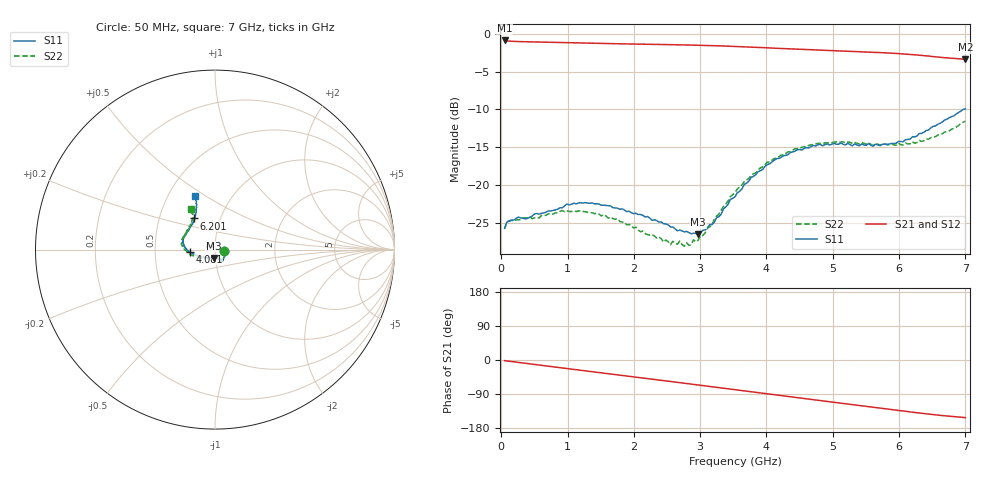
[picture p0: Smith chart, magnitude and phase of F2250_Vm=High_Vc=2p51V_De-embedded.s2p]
! Integrated Device Technology
! Corporate Headquarters
! 6024 Silver Creek Valley Road
! San Jose, CA 95138  USA
! Phone:  1-408-284-8200
! Toll Free:  1-800-223-1366
! Webpage:  http://www.idt.com/
! Timing and RF Division
! 515 Groton Road, Suite 102
! Westford, MA 01886-6024
! Device:  F2250
! Description: Voltage Variable RF Attenuator
! Frequency:  50.0 -  6000.00 MHz
! Package:  3x3 mm Thin QFN Plastic Package: 16 pin
! Ports:  2 RF, 3 DC
!  Pin  1  = GND
!  Pin  2  = NC
!  Pin  3  = RF1  = Port 1
!  Pin  4  = NC
!  Pin  5  = GND
!  Pin  6  = GND
!  Pin  7  = GND
!  Pin  8  = GND
!  Pin  9  = NC
!  Pin 10  = RF2  = Port 2
!  Pin 11  = NC
!  Pin 12  = GND
!  Pin 13  = GND
!  Pin 14  = VCNTRL
!  Pin 15  = VDD
!  Pin 16  = VMODE
! Vcntrl:  2.510 Volts
! Vmode:  +3.300 Volts
! Vdd:  +3.30  Volts
! Current:  1.314 mA
! Data:  The device was measured on a the F2250 evaluation board which has
!  individual transmission lines to the RF pins.  Data was collected
!  using a calibrated network analyzer.  The evaluation board was
!  de-embedded using a TRL calibration technique.
!  The reference plane is the edge of the package pin.
! Misc:  SN 10
!  Action Tracker AT0258
! Date Measured:  2014-11-26
! Date:  2015-10-15  MJV
! Note:
!  Integrated Device Technology supplies this data as a sample of measured
!  data at the package pin for this product.  Your particular data for this
!  product may vary.
!  Data was taken at 25 degrees C.
!  Integrated Device Technology reserves the right to change this data at anytime.
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# GHz S dB R 50
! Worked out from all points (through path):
!   201 points, 50 MHz to 7 GHz, reference 50 ohm
!   highest |S21| = -0.89 dB at 50 MHz (marker M1); lowest = -3.4 dB at 7 GHz (marker M2)
!   group delay of S21, straight-line fit = 61.2 ps
!   lowest |S11| = -26.5 dB at 2.969 GHz (marker M3), VSWR 1.10, Z = 49.1 - j4.62 ohm
!   |S11| at or under -10 dB: start of sweep to 6.967 GHz
!   |S22| runs from -28.1 to -11.6 dB; largest |S21 - S12| = 0.002
!   S11 on the Smith chart (normalised r, x): 50 MHz: 1.11, -0.02; 4.081 GHz: 0.75, -0.02; 6.201 GHz: 0.75, +0.27; 7 GHz: 0.68, +0.45
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0.05  -25.65 -10.7  -0.89 -1.8  -0.89 -1.8  -25.82 -10.9
0.1195  -24.75 -10.3  -0.98 -3.2  -0.98 -3.2  -24.68 -8.9
0.57125  -23.83 -31.3  -1.10 -13.3  -1.10 -13.3  -24.33 -31.4
0.91875  -23.00 -50.1  -1.17 -21.0  -1.17 -21.1  -23.35 -51.0
1.2315  -22.36 -57.9  -1.24 -27.9  -1.24 -27.9  -23.47 -61.6
1.75275  -23.04 -64.9  -1.33 -39.1  -1.33 -39.1  -24.42 -67.8
2.37825  -24.87 -64.5  -1.42 -52.8  -1.42 -52.8  -26.87 -66.8
2.552  -25.51 -69.5  -1.44 -56.7  -1.44 -56.7  -27.86 -73.2
2.691  -25.93 -77.5  -1.47 -59.8  -1.47 -59.8  -27.37 -80.9
2.7605  -26.17 -79.7  -1.48 -61.3  -1.48 -61.3  -28.05 -85.4
2.969  -26.49 -97.8  -1.52 -66.0  -1.52 -66.0  -27.28 -105.0
3.1775  -25.21 -120.8  -1.57 -70.7  -1.57 -70.7  -25.24 -126.9
3.525  -21.53 -152.8  -1.68 -78.5  -1.68 -78.6  -20.97 -148.8
3.76825  -18.97 -164.8  -1.77 -84.0  -1.77 -84.1  -18.70 -159.8
4.081  -16.95 -175.7  -1.90 -91.0  -1.90 -91.0  -16.72 -171.5
4.4285  -15.54 176.0  -2.03 -98.6  -2.03 -98.6  -15.20 178.6
4.7065  -14.76 169.1  -2.13 -104.8  -2.13 -104.8  -14.69 172.9
5.054  -14.60 160.9  -2.26 -112.5  -2.26 -112.5  -14.29 165.9
5.85325  -14.56 135.1  -2.56 -130.0  -2.56 -130.1  -14.69 147.2
6.20075  -13.62 123.6  -2.77 -137.7  -2.77 -137.8  -14.27 138.2
6.54825  -12.18 115.6  -3.04 -144.7  -3.04 -144.9  -13.60 126.8
7  -9.91 110.8  -3.37 -152.1  -3.38 -152.2  -11.56 120.6
